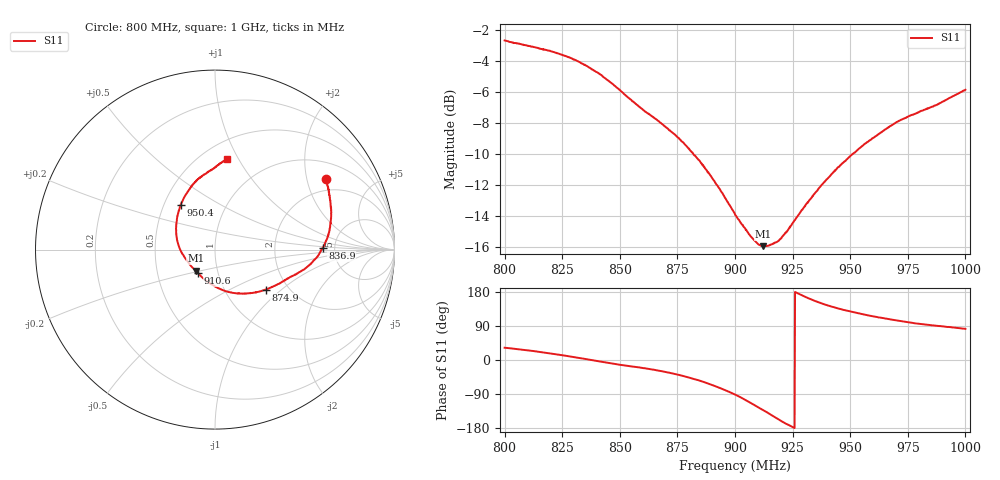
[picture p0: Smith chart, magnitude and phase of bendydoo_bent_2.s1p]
# HZ S RI R 50
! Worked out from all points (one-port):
!   1010 points, 800 MHz to 1 GHz, reference 50 ohm
!   lowest |S11| = -15.9 dB at 912.2 MHz (marker M1), VSWR 1.38, Z = 39.3 - j9.52 ohm
!   |S11| at or under -10 dB: 882 MHz to 951 MHz (69.09 MHz wide, 7.54 % of centre)
!   S11 on the Smith chart (normalised r, x): 800 MHz: 1.54, +2.63; 836.9 MHz: 3.99, +0.12; 874.9 MHz: 1.54, -0.79; 910.6 MHz: 0.80, -0.21; 950.4 MHz: 0.61, +0.34; 1 GHz: 0.66, +0.90
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8e8  0.6199 0.3929
8.126858e8  0.641 0.2786
8.186323e8  0.647 0.2155
8.251734e8  0.644 0.1431
8.313181e8  0.6272 0.0708
8.368682e8  0.5993 0.01
8.4222e8  0.5643 -0.0468
8.501486e8  0.4952 -0.1114
8.677899e8  0.3486 -0.1937
8.749256e8  0.2814 -0.2237
8.751239e8  0.28 -0.2232
8.81665e8  0.2076 -0.2416
8.888008e8  0.1235 -0.2442
8.941526e8  0.0592 -0.2315
9.000991e8  -0.00393 -0.2016
9.066402e8  -0.0667 -0.1592
9.106045e8  -0.0961 -0.1297
9.121903e8  -0.1078 -0.1182
9.189296e8  -0.1531 -0.0658
9.250743e8  -0.1898 -0.00917
9.304261e8  -0.2093 0.0491
9.359762e8  -0.2166 0.1107
9.423191e8  -0.2113 0.1756
9.500495e8  -0.1926 0.2453
9.504459e8  -0.1917 0.2484
9.631318e8  -0.1377 0.3441
9.750247e8  -0.0704 0.4114
9.999999e8  0.0693 0.5047
